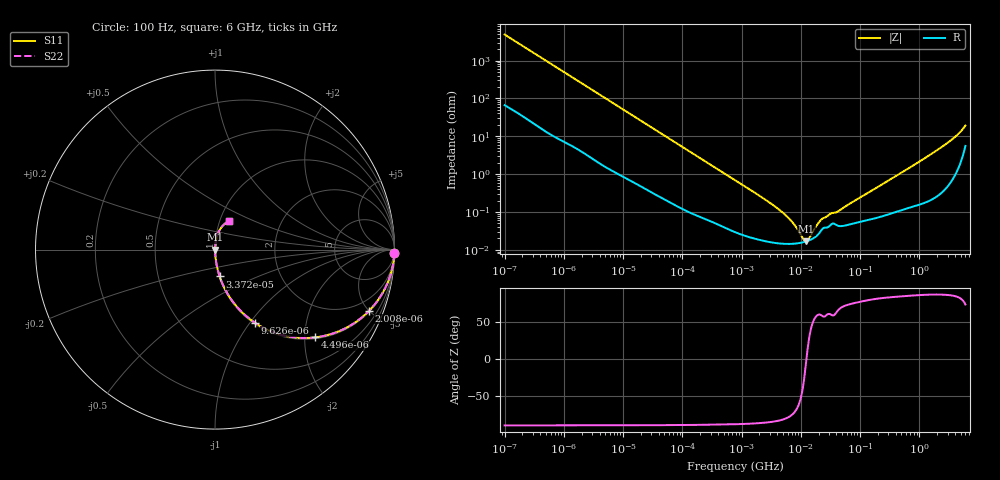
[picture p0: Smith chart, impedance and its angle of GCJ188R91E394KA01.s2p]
!Murata Part Number: GCJ188R91E394KA01
!These Parameters are Measured in Series Mode Connection
!Data Generated on Mar 13, 2026
!  o--ll--o
!Port1  Port2
!  o------o
!Operation Temp=25[degC], DC Bias Voltage=0[V]
!Freq. Start=100[Hz] Stop=6[GHz] 401[Steps]
# Hz S RI R 50
!Freq.(Hz) S11(Real) S11(Imag) S21(Real) S21(Imag) S12(Real) S12(Imag) S22(Real) S22(Imag)
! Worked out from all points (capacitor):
!   401 points, 100 Hz to 6 GHz, reference 50 ohm
!   read as one part in series: C = 323 nF near 109 Hz
!   lowest |Z| = 16.7 mohm at 12.44 MHz (marker M1)
!   series resonance near 12.45 MHz, so ESL is about 510 pH
!   S11 on the Smith chart (normalised r, x): 100 Hz: 2, -98; 2.008 kHz: 1.08, -5.02; 4.496 kHz: 1.03, -2.26; 9.626 kHz: 1.02, -1.06; 33.72 kHz: 1.01, -0.31; 6 GHz: 1.11, +0.37
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100  0.9993 -0.0204  0.000692 0.0204  0.000692 0.0204  0.9993 -0.0204
548  0.9866 -0.1085  0.0134 0.1085  0.0134 0.1085  0.9866 -0.1085
1174  0.945 -0.2207  0.055 0.2207  0.055 0.2207  0.945 -0.2207
2008  0.859 -0.3403  0.141 0.3403  0.141 0.3403  0.859 -0.3403
4496  0.5595 -0.4889  0.4405 0.4889  0.4405 0.4889  0.5595 -0.4889
9626  0.2238 -0.4085  0.7762 0.4085  0.7762 0.4085  0.2238 -0.4085
16473  0.0929 -0.2815  0.9071 0.2815  0.9071 0.2815  0.0929 -0.2815
33721  0.0259 -0.1493  0.9741 0.1493  0.9741 0.1493  0.0259 -0.1493
40335  0.0187 -0.126  0.9813 0.126  0.9813 0.126  0.0187 -0.126
129199  0.00264 -0.0406  0.9974 0.0406  0.9974 0.0406  0.00264 -0.0406
774597  0.000341 -0.00698  0.9997 0.00698  0.9997 0.00698  0.000341 -0.00698
4856642  0.000146 -0.000974  0.9999 0.000974  0.9999 0.000974  0.000146 -0.000974
6948629  0.000144 -0.000554  0.9999 0.000554  0.9999 0.000554  0.000144 -0.000554
1.087309e7  0.000158 -0.000122  0.9998 0.000122  0.9998 0.000122  0.000158 -0.000122
1.243624e7  0.000167 -1.1e-06  0.9998 1.1e-06  0.9998 1.1e-06  0.000167 -1.1e-06
1.555665e7  0.000193 0.000204  0.9998 -0.000204  0.9998 -0.000204  0.000193 0.000204
1.946e7  0.000251 0.000423  0.9997 -0.000423  0.9997 -0.000423  0.000251 0.000423
2.327686e7  0.00036 0.000565  0.9996 -0.000565  0.9996 -0.000565  0.00036 0.000565
4.35672e7  0.000427 0.000972  0.9996 -0.000972  0.9996 -0.000972  0.000427 0.000972
3.124326e8  0.000924 0.00692  0.9991 -0.00692  0.9991 -0.00692  0.000924 0.00692
2.450438e9  0.00615 0.0529  0.9938 -0.0529  0.9938 -0.0529  0.00615 0.0529
6e9  0.0806 0.1604  0.9194 -0.1604  0.9194 -0.1604  0.0806 0.1604
